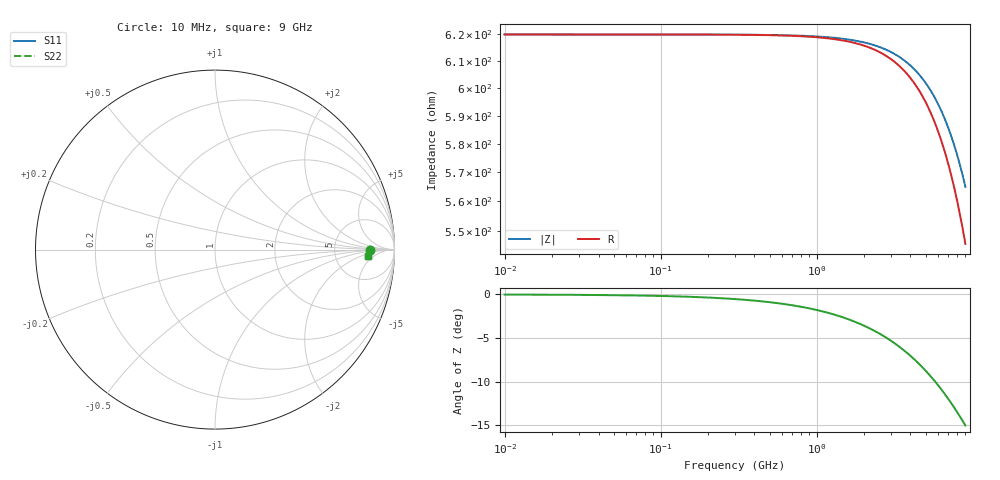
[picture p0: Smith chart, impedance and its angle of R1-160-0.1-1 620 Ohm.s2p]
!version-1
!date-03.2021
# MHz S RI R 50
!Freq ReS11 ImS11 ReS21 ImS21 ReS12 ImS12 ReS22 ImS22
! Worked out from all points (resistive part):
!   451 points, 10 MHz to 9 GHz, reference 50 ohm
!   read as one part in series: R = 620 ohm at 50 MHz
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10  0.8611 -3.73e-05  0.1389 3.73e-05  0.1389 3.73e-05  0.8611 -3.75e-05
370  0.8611 -0.00138  0.1389 0.00138  0.1389 0.00138  0.8611 -0.00139
750  0.8611 -0.0028  0.1389 0.00279  0.1389 0.00279  0.8611 -0.00281
1130  0.861 -0.00421  0.139 0.00421  0.139 0.00421  0.861 -0.00424
1510  0.8609 -0.00563  0.1391 0.00563  0.1391 0.00563  0.8609 -0.00566
1870  0.8608 -0.00697  0.1392 0.00697  0.1392 0.00697  0.8608 -0.00701
2250  0.8606 -0.00839  0.1394 0.00838  0.1394 0.00838  0.8606 -0.00843
2630  0.8604 -0.0098  0.1396 0.0098  0.1396 0.0098  0.8604 -0.00986
3010  0.8602 -0.0112  0.1398 0.0112  0.1398 0.0112  0.8602 -0.0113
3370  0.86 -0.0126  0.14 0.0126  0.14 0.0126  0.86 -0.0126
3750  0.8597 -0.014  0.1403 0.014  0.1403 0.014  0.8597 -0.014
4130  0.8594 -0.0154  0.1406 0.0154  0.1406 0.0154  0.8594 -0.0155
4510  0.859 -0.0168  0.141 0.0168  0.141 0.0168  0.859 -0.0169
4870  0.8587 -0.0181  0.1413 0.0181  0.1413 0.0181  0.8587 -0.0182
5250  0.8583 -0.0195  0.1417 0.0195  0.1417 0.0195  0.8583 -0.0197
5630  0.8579 -0.021  0.1421 0.021  0.1421 0.021  0.8579 -0.0211
6010  0.8574 -0.0224  0.1426 0.0224  0.1426 0.0224  0.8574 -0.0225
6750  0.8564 -0.0251  0.1436 0.0251  0.1436 0.0251  0.8564 -0.0253
7130  0.8559 -0.0265  0.1441 0.0265  0.1441 0.0265  0.8559 -0.0267
7510  0.8553 -0.0279  0.1447 0.0279  0.1447 0.0279  0.8553 -0.0281
8190  0.8542 -0.0304  0.1458 0.0304  0.1458 0.0304  0.8542 -0.0306
9000  0.8527 -0.0334  0.1473 0.0334  0.1473 0.0334  0.8527 -0.0336
